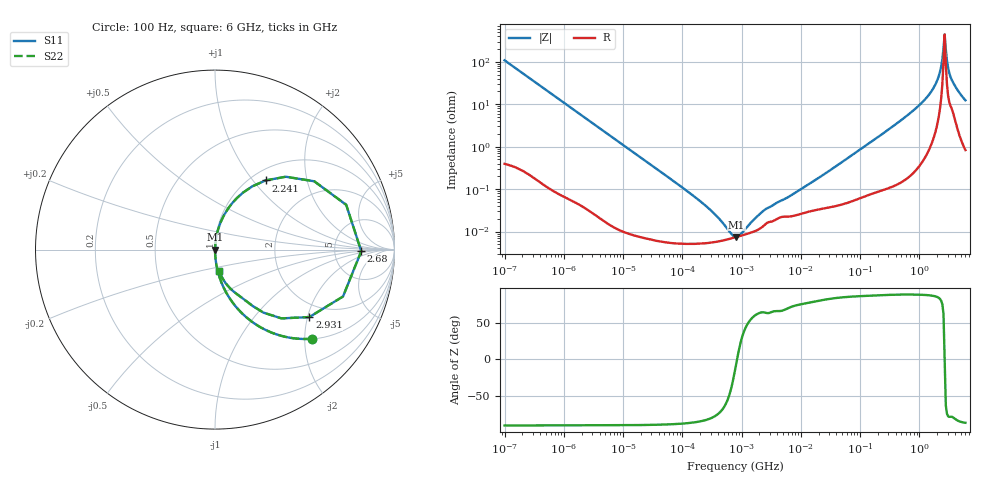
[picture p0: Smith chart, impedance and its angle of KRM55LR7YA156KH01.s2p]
!Murata Part Number: KRM55LR7YA156KH01
!These Parameters are Measured in Series Mode Connection
!Data Generated on Jan 08, 2026
!  o--ll--o
!Port1  Port2
!  o------o
!Operation Temp=25[degC], DC Bias Voltage=0[V]
!Freq. Start=100[Hz] Stop=6[GHz] 401[Steps]
# Hz S RI R 50
!Freq.(Hz) S11(Real) S11(Imag) S21(Real) S21(Imag) S12(Real) S12(Imag) S22(Real) S22(Imag)
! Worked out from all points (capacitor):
!   401 points, 100 Hz to 6 GHz, reference 50 ohm
!   read as one part in series: C = 14.7 uF near 109 Hz
!   lowest |Z| = 7.47 mohm at 810.1 kHz (marker M1)
!   series resonance near 838.7 kHz, so ESL is about 2.5 nH
!   S11 on the Smith chart (normalised r, x): 100 Hz: 1.01, -2.17; 2.241 GHz: 1.16, +1.16; 2.68 GHz: 9.78, -0.52; 2.931 GHz: 1.59, -2.05; 6 GHz: 1.02, -0.25
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100  0.5396 -0.4966  0.4604 0.4966  0.4604 0.4966  0.5396 -0.4966
335  0.0966 -0.2928  0.9034 0.2928  0.9034 0.2928  0.0966 -0.2928
2008  0.00336 -0.0543  0.9966 0.0543  0.9966 0.0543  0.00336 -0.0543
40335  6.66e-05 -0.00273  0.9999 0.00273  0.9999 0.00273  6.66e-05 -0.00273
241822  5.32e-05 -0.000414  0.9999 0.000414  0.9999 0.000414  5.32e-05 -0.000414
619225  6.7e-05 -7.65e-05  0.9999 7.65e-05  0.9999 7.65e-05  6.7e-05 -7.65e-05
774597  7.29e-05 -1.93e-05  0.9999 1.93e-05  0.9999 1.93e-05  7.29e-05 -1.93e-05
810067  7.42e-05 -8.4e-06  0.9999 8.4e-06  0.9999 8.4e-06  7.42e-05 -8.4e-06
1059725  8.25e-05 5.64e-05  0.9999 -5.64e-05  0.9999 -5.64e-05  8.25e-05 5.64e-05
2481164  0.000146 0.000295  0.9999 -0.000295  0.9999 -0.000295  0.000146 0.000295
1.555665e7  0.00031 0.00144  0.9997 -0.00144  0.9997 -0.00144  0.00031 0.00144
3.124326e8  0.00175 0.0261  0.9982 -0.0261  0.9982 -0.0261  0.00175 0.0261
8.749838e8  0.00909 0.0791  0.9909 -0.0791  0.9909 -0.0791  0.00909 0.0791
1.565993e9  0.0449 0.1814  0.9551 -0.1814  0.9551 -0.1814  0.0449 0.1814
1.95892e9  0.121 0.2862  0.879 -0.2862  0.879 -0.2862  0.121 0.2862
2.240541e9  0.2821 0.3856  0.7179 -0.3856  0.7179 -0.3856  0.2821 0.3856
2.450438e9  0.5531 0.3805  0.4469 -0.3805  0.4469 -0.3805  0.5531 0.3805
2.679998e9  0.8148 -0.00895  0.1852 0.00895  0.1852 0.00895  0.8148 -0.00895
2.931063e9  0.5258 -0.3758  0.4742 0.3758  0.4742 0.3758  0.5258 -0.3758
3.205649e9  0.2699 -0.3509  0.7301 0.3509  0.7301 0.3509  0.2699 -0.3509
3.666503e9  0.1445 -0.2645  0.8555 0.2645  0.8555 0.2645  0.1445 -0.2645
6e9  0.0229 -0.1196  0.9771 0.1196  0.9771 0.1196  0.0229 -0.1196
